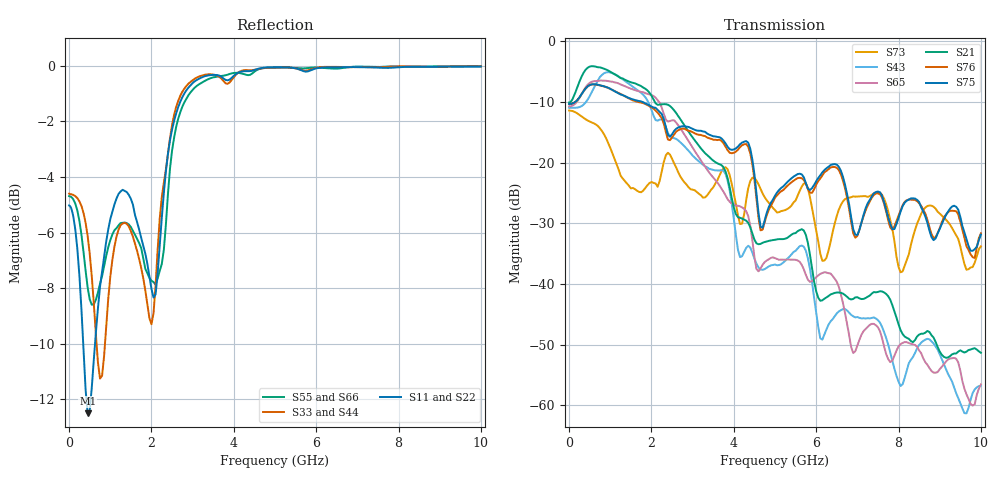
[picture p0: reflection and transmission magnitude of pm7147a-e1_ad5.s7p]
# GHz S DB R 50
! S-Parameters data
! Freq  dbS11  angS11  dbS12  angS12  dbS13  angS13  dbS14  angS14
!  dbS15  angS15  dbS16  angS16  dbS17  angS17  dbS21  angS21
!  dbS22  angS22  dbS23  angS23  dbS24  angS24  dbS25  angS25
!  dbS26  angS26  dbS27  angS27  dbS31  angS31  dbS32  angS32
!  dbS33  angS33  dbS34  angS34  dbS35  angS35  dbS36  angS36
!  dbS37  angS37  dbS41  angS41  dbS42  angS42  dbS43  angS43
!  dbS44  angS44  dbS45  angS45  dbS46  angS46  dbS47  angS47
!  dbS51  angS51  dbS52  angS52  dbS53  angS53  dbS54  angS54
!  dbS55  angS55  dbS56  angS56  dbS57  angS57  dbS61  angS61
!  dbS62  angS62  dbS63  angS63  dbS64  angS64  dbS65  angS65
!  dbS66  angS66  dbS67  angS67  dbS71  angS71  dbS72  angS72
!  dbS73  angS73  dbS74  angS74  dbS75  angS75  dbS76  angS76
!  dbS77  angS77
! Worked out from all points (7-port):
!   279 points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, 1 Hz to 10 GHz, reference 50 ohm
!   strongest paths, dB at 1 Hz, 7.943 MHz, 3.05 GHz, 6.55 GHz, 10 GHz:
!     S75: -10.3, -10.3, -14.6, -20.7, -31.9
!     S76: -10.3, -10.3, -15.2, -21.2, -31.7
!     S21: -10.1, -10.1, -16.3, -41.4, -51.3
!     S65: -10.7, -10.7, -18.1, -40.5, -56.6
!     S43: -11.0, -11.0, -19.2, -44.5, -56.8
!     S73: -11.4, -11.4, -24.6, -27.8, -33.8
!   lowest |S11| = -12.5 dB at 450 MHz (marker M1), VSWR 1.62, Z = 30.9 + j1.24 ohm
!   |S11| at or under -10 dB: 342.2 MHz to 629 MHz (286.8 MHz wide, 59.1 % of centre)
